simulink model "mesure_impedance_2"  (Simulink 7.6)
settings: Solver=ode23tb  SolverMode=SingleTasking  StartTime=0.0  StopTime=0.05  RelTol=1e-4
StopFcn:
  | close all
  | load phasor.mat
  | plotyy(x(1,:),x(2,:), x(1,:),x(3,:))
  | grid
  | title('Tracé des phaseurs, courant de charge et Tension en bout de ligne')
  | xlabel('temps')
libraries: powerlib x11

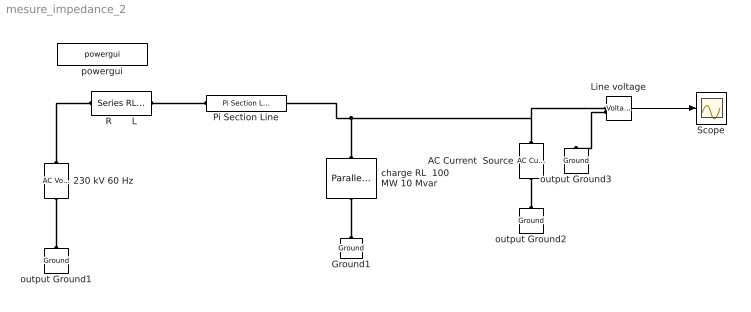
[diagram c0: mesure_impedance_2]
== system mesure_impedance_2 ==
  230 kV 60 Hz : powerlib/Electrical Sources/AC Voltage Source  Description=source block  DialogController=POWERSYS.PowerSysDialog  SystemSampleTime=-1  Amplitude=230e3  Phase=0  Frequency=60  SampleTime=0  Measurements=None
  AC Current  Source : powerlib/Electrical Sources/AC Current Source  DialogController=POWERSYS.PowerSysDialog  SystemSampleTime=-1  Amplitude=0  Phase=0  Frequency=60  SampleTime=0  Measurements=None
  Ground1 : powerlib/Elements/Ground  DialogController=POWERSYS.PowerSysDialog  PhysicalDomain=powersysdomain  SubClassName=unknown  LeftPortType=p1  RightPortType=p1  LConnTagsString=a
  Line voltage : powerlib/Measurements/Voltage Measurement  Tag=PoWeRsYsTeMmEaSuReMeNt  DialogController=POWERSYS.PowerSysDialog  SystemSampleTime=-1  PhasorSimulation=off  OutputType=Magnitude  PSBequivalent=0
  Pi Section Line : powerlib/Elements/Pi Section Line  DialogController=POWERSYS.PowerSysDialog  PhysicalDomain=powersysdomain  SubClassName=unknown  LeftPortType=p1  RightPortType=p1  LConnTagsString=__new0  RConnTagsString=__new0  Frequency=60  Resistance=0.2568  Inductance=2e-3  Capacitance=8.6e-9  Length=100  PiSections=1  Measurements=None
  R       L : powerlib/Elements/Series RLC Branch  DialogController=POWERSYS.PowerSysDialog  PhysicalDomain=powersysdomain  SubClassName=unknown  LeftPortType=p1  RightPortType=p1  LConnTagsString=__new0  RConnTagsString=__new0  BranchType=RL  Resistance=3  Inductance=1e-2  SetiL0=off  InitialCurrent=0  Capacitance=[]  Setx0=off  InitialVoltage=0  Measurements=None
  Scope : Scope
  charge RL  100 MW 10 Mvar : powerlib/Elements/Parallel RLC Load  DialogController=POWERSYS.PowerSysDialog  PhysicalDomain=powersysdomain  SubClassName=unknown  LeftPortType=p1  RightPortType=p1  LConnTagsString=a  RConnTagsString=__new0  NominalVoltage=230/sqrt(2)  NominalFrequency=60  ActivePower=100e6  InductivePower=10e6  CapacitivePower=0  Setx0=off  InitialVoltage=0  SetiL0=off  InitialCurrent=0  Measurements=None
  output Ground1 : powerlib/Elements/Ground  DialogController=POWERSYS.PowerSysDialog  PhysicalDomain=powersysdomain  SubClassName=unknown  LeftPortType=p1  RightPortType=p1  LConnTagsString=a
  output Ground2 : powerlib/Elements/Ground  DialogController=POWERSYS.PowerSysDialog  PhysicalDomain=powersysdomain  SubClassName=unknown  LeftPortType=p1  RightPortType=p1  LConnTagsString=a
  output Ground3 : powerlib/Elements/Ground  DialogController=POWERSYS.PowerSysDialog  PhysicalDomain=powersysdomain  SubClassName=unknown  LeftPortType=p1  RightPortType=p1  LConnTagsString=a
  powergui : powerlib/powergui  Priority=2  SystemSampleTime=-1  SimulationMode=Continuous  SampleTime=0  frequency=60  SPID=off  DisableSnubberDevices=off  DisableRonSwitches=off  DisableVfSwitches=off  SwTol=0  Interpol=off  frequencyindice=60  echomessages=off  HookPort=off  DisplayEquations=off  FunctionMessages=off  EnableUseOfTLC=off  x0status=blocks  RestoreLinks=warning  ResistiveCurrentMeasurement=off  Frange=0:200  Ylog=off  Xlog=off  ShowGrid=on  save=off  variable=ZData  ZoomFFT=on  StartTime=0.0  cycles=1  DisplayStyle=off  fundamental=60  FreqAxis=off  MaxFrequency=1000  frequencyindicesteady=1  RmsSteady=1  display=off  Ts=0  methode=off
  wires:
  Line voltage/1 -> Scope/1
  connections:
  charge RL  100 MW 10 Mvar/RConn1 -- Ground1/LConn1
  230 kV 60 Hz/RConn1 -- R       L/LConn1
  output Ground1/LConn1 -- 230 kV 60 Hz/LConn1
  AC Current  Source/RConn1 -- Pi Section Line/RConn1 -- charge RL  100 MW 10 Mvar/LConn1 -- Line voltage/LConn1
  Pi Section Line/LConn1 -- R       L/RConn1
  AC Current  Source/LConn1 -- output Ground2/LConn1
  Line voltage/LConn2 -- output Ground3/LConn1
